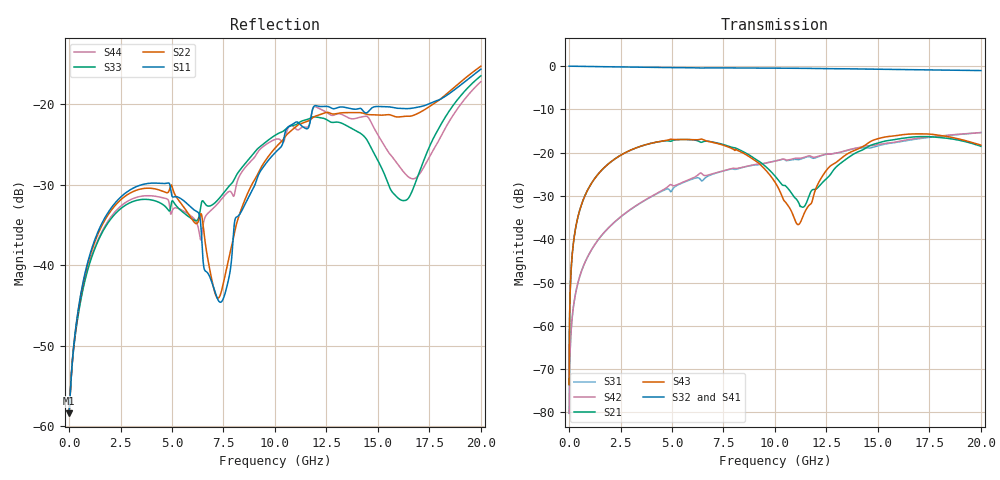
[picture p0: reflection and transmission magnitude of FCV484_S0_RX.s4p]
! Touchstone generated by fitter/viewer
# HZ S  RI R 5.000000e+001
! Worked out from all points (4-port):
!   4999 points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, 4.001 MHz to 20 GHz, reference 50 ohm
!   strongest paths, dB at 4.001 MHz, 5.001 GHz, 10 GHz, 15 GHz, 20 GHz:
!     S32: 0.0, -0.4, -0.5, -0.7, -1.0
!     S41: 0.0, -0.4, -0.5, -0.7, -1.0
!     S43: -73.6, -16.9, -26.8, -16.8, -18.2
!     S21: -73.6, -17.2, -25.4, -17.8, -18.5
!     S42: -80.2, -27.5, -21.9, -18.1, -15.4
!     S31: -80.2, -28.7, -21.9, -18.4, -15.3
!   lowest |S11| = -58.4 dB at 4.001 MHz (marker M1), VSWR 1.00, Z = 50.1 + j0.00725 ohm
!   |S11| at or under -10 dB: start of sweep to end of sweep
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4000800  0.0012 7.23e-05  8.6e-05 0.000192  -8.46e-05 -4.89e-05  0.9988 -0.00136
         8.6e-05 0.000192  0.00121 7.51e-05  0.9988 -0.00137  -8.46e-05 -4.89e-05
         -8.46e-05 -4.89e-05  0.9988 -0.00137  0.00121 7.58e-05  8.6e-05 0.000192
         0.9988 -0.00136  -8.46e-05 -4.89e-05  8.6e-05 0.000192  0.0012 7.3e-05
5.521104e8  0.00395 -0.00507  0.00441 0.0226  -0.00101 -0.00381  0.9794 -0.1648
            0.00441 0.0226  0.004 -0.00487  0.9792 -0.1657  -0.000997 -0.00381
            -0.00101 -0.00381  0.9792 -0.1657  0.0038 -0.00451  0.00439 0.0226
            0.9794 -0.1648  -0.000997 -0.00381  0.00439 0.0226  0.00372 -0.00471
2.860572e9  -0.0126 -0.0259  0.0773 0.0688  -0.0143 -0.0154  0.6525 -0.7252
            0.0773 0.0688  -0.012 -0.0248  0.6488 -0.7285  -0.0141 -0.0157
            -0.0143 -0.0154  0.6488 -0.7285  -0.0105 -0.0217  0.0774 0.069
            0.6525 -0.7252  -0.0141 -0.0157  0.0774 0.069  -0.0116 -0.0222
7.373475e9  -0.000526 -0.00588  0.1131 -0.0567  -0.0515 0.0316  -0.5003 -0.813
            0.1131 -0.0567  0.000504 -0.00669  -0.5092 -0.8072  -0.0509 0.033
            -0.0515 0.0316  -0.5092 -0.8072  -0.0039 -0.0265  0.1033 -0.0694
            -0.5003 -0.813  -0.0509 0.033  0.1033 -0.0694  -0.00499 -0.0249
1.087017e10  0.0349 -0.0666  0.0253 -0.0201  0.00473 0.0832  -0.9411 -0.0126
             0.0253 -0.0201  0.0293 -0.0633  -0.9449 0.00341  0.00375 0.085
             0.00473 0.0832  -0.9449 0.00341  -0.0364 -0.0641  -0.017 -0.00903
             -0.9411 -0.0126  0.00375 0.085  -0.017 -0.00903  -0.0362 -0.0633
1.567113e10  -0.00359 -0.0955  0.14 8.59e-05  0.1268 0.0241  -0.1949 0.8942
             0.14 8.59e-05  -0.00331 -0.085  -0.1631 0.8995  0.1284 0.022
             0.1268 0.0241  -0.1631 0.8995  -0.0154 0.0242  0.1458 0.0527
             -0.1949 0.8942  0.1284 0.022  0.1458 0.0527  -0.0316 0.0354
2e10  0.0392 -0.1599  0.0651 -0.099  0.0659 -0.1577  0.771 0.4477
      0.0651 -0.099  0.0394 -0.1673  0.7861 0.4146  0.0607 -0.1594
      0.0659 -0.1577  0.7861 0.4146  0.0561 -0.1388  0.0112 -0.122
      0.771 0.4477  0.0607 -0.1594  0.0112 -0.122  0.059 -0.1245
